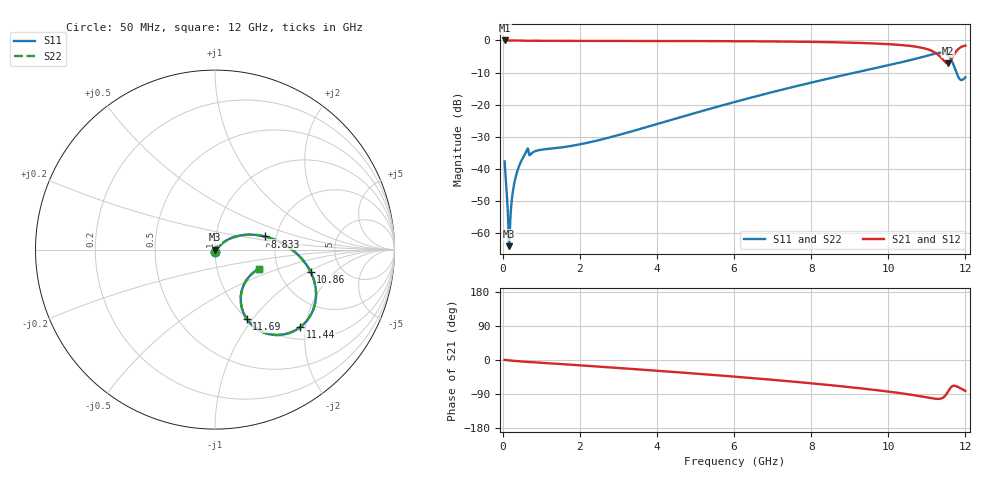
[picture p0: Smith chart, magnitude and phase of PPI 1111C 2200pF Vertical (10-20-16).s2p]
# GHz S MA R 50
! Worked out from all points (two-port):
!   1601 points, 50 MHz to 12 GHz, reference 50 ohm
!   highest |S21| = 0.00 dB at 57.47 MHz (marker M1); lowest = -7.1 dB at 11.54 GHz (marker M2)
!   |S21| within 3 dB of the highest: start of sweep to 11.08 GHz; 11.79 GHz to end of sweep
!   lowest |S11| = -64.0 dB at 169.5 MHz (marker M3), VSWR 1.00, Z = 50.1 + j0.0046 ohm
!   |S11| at or under -10 dB: start of sweep to 9.134 GHz; 11.77 GHz to end of sweep
!   |S22| runs from -64.0 to -3.8 dB; largest |S21 - S12| = 0
!   S11 on the Smith chart (normalised r, x): 50 MHz: 1.00, -0.03; 8.833 GHz: 1.75, +0.28; 10.86 GHz: 3.00, -1.08; 11.44 GHz: 1.27, -1.87; 11.69 GHz: 0.99, -0.94; 12 GHz: 1.60, -0.37
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0.05  0.01318 -88.0  0.9995 0.4  0.9995 0.4  0.01318 -88.0
0.05746875  0.01113 -87.8  0.9995 0.3  0.9995 0.3  0.01113 -87.8
0.1321563  0.002217 -76.6  0.9994 -0.7  0.9994 -0.7  0.002217 -76.6
0.1695  0.0006344 4.2  0.9994 -1.1  0.9994 -1.1  0.0006344 4.2
0.2068437  0.00203 66.7  0.9992 -1.5  0.9992 -1.5  0.00203 66.7
0.2665938  0.0046 74.4  0.9989 -2.0  0.9989 -2.0  0.0046 74.4
0.3412812  0.007698 73.5  0.9981 -2.7  0.9981 -2.7  0.007698 73.5
0.4458437  0.01195 67.7  0.9961 -3.6  0.9961 -3.6  0.01195 67.7
0.6101562  0.01869 53.5  0.99 -4.9  0.99 -4.9  0.01869 53.5
2.044156  0.02456 33.5  0.9832 -14.3  0.9832 -14.3  0.02456 33.5
4.038312  0.0509 40.8  0.9807 -28.6  0.9807 -28.6  0.0509 40.8
6.025  0.1109 35.3  0.9732 -44.0  0.9732 -44.0  0.1109 35.3
8.019156  0.2225 21.9  0.9501 -61.7  0.9501 -61.7  0.2225 21.9
8.83325  0.2882 14.7  0.93 -69.8  0.93 -69.8  0.2882 14.7
10.01331  0.4137 1.6  0.8747 -83.5  0.8747 -83.5  0.4137 1.6
10.86475  0.5482 -13.3  0.7707 -96.2  0.7707 -96.2  0.5482 -13.3
11.23819  0.6293 -27.2  0.6329 -102.4  0.6329 -102.4  0.6293 -27.2
11.43984  0.642 -42.2  0.4853 -97.9  0.4853 -97.9  0.642 -42.2
11.53694  0.5992 -52.4  0.4416 -85.2  0.4416 -85.2  0.5992 -52.4
11.68631  0.4252 -65.4  0.5746 -68.1  0.5746 -68.1  0.4252 -65.4
11.85063  0.2517 -49.7  0.764 -73.5  0.764 -73.5  0.2517 -49.7
12  0.2681 -23.5  0.8314 -81.5  0.8314 -81.5  0.2681 -23.5
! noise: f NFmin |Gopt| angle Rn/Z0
0.05  0.0004133  0.8786  0.333  0.0007363
1.372  0.01441  0.9037  8.936  0.03258
2.701  0.02056  0.8713  17.47  0.03363
4.031  0.02562  0.8514  25.78  0.03492
5.36  0.03039  0.8398  33.78  0.03682
6.682  0.03523  0.835  41.38  0.03953
8.012  0.04067  0.8364  48.63  0.04372
9.341  0.04813  0.8462  55.47  0.05219
10.67  0.07086  0.8847  62  0.09816
12  0.1169  0.9242  68.32  0.2341
